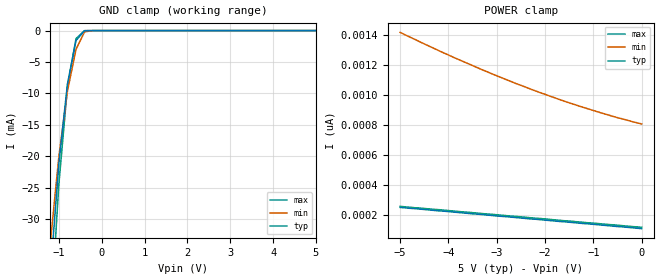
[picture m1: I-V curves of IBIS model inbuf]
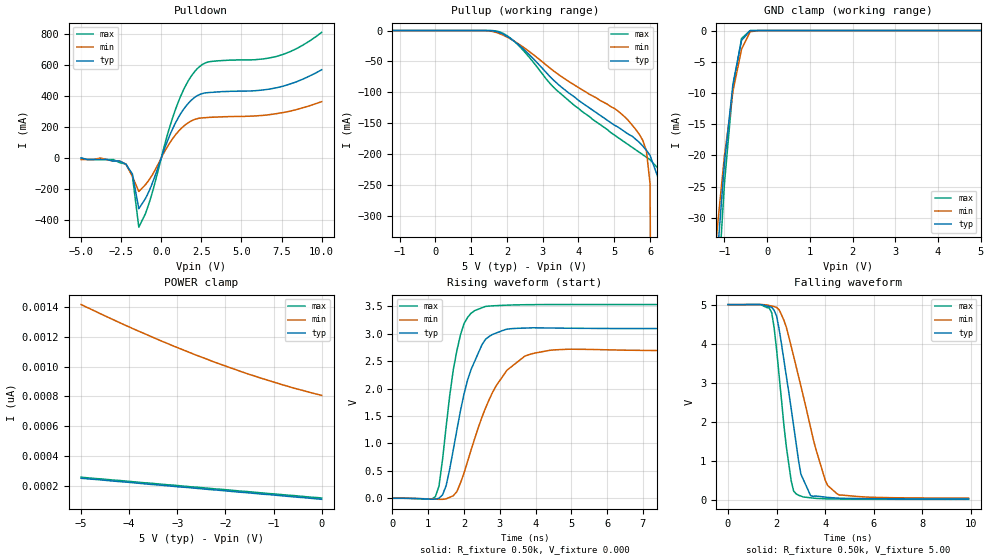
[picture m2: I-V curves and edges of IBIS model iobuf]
| IBIS file 61501n.ibs created by s2ibis2 version 1.0
| North Carolina State University Electronics Research Laboratory  1995
[IBIS ver]   2.1
[File name]   61501n.ibs
[File Rev]   0.1
[Date]   Tuesday, June 10, 1997
[Source]   IDT
[Notes]   1. Temp typ=25C, min=100C, max=0C 2. Ramp rates based on 500
   ohm load
[Copyright]   Copyright 1997, Integrated Device Technology, Inc.
[Disclaimer] Integrated Device Technology, Inc. ("IDT") hereby grants the
   user of this IBIS model a non-exclusive, nontransferable
   license to use this IBIS model under the following terms.
   The user is granted this license only to use the IBIS model
   and is not granted rights to sell, copy (except as needed to
   run the IBIS model), rent, lease or sub-license the IBIS model
   in whole or in part, or in modified form to anyone.
   The User may modify the IBIS model to suit its specific
   applications, but rights to derivative works and such
   modifications shall belong to IDT.
   This IBIS model is provided on an "AS IS" basis and IDT
   makes absolutely no warranty with respect to the information
   contained herein. IDT DISCLAIMS AND CUSTOMER WAIVES ALL
   WARRANTIES, EXPRESS AND IMPLIED, INCLUDING WARRANTIES OF
   MERCHANTABILITY AND FITNESS FOR A PARTICULAR PURPOSE. THE
   ENTIRE RISK AS TO QUALITY AND PERFORMANCE IS WITH THE
   USER ACCORDINGLY, IN NO EVENT SHALL IDT BE LIABLE
   FOR ANY DIRECT OR INDIRECT DAMAGES, WHETHER IN CONTRACT OR
   TORT, INCLUDING ANY LOST PROFITS OR OTHER INCIDENTAL,
   CONSEQUENTIAL, EXEMPLARY, OR PUNITIVE DAMAGES ARISING OUT OF
   THE USE OR APPLICATION OF THE IBIS model.  Further, IDT
   reserves the right to make changes without notice to any
   product herein to improve reliability, function, or design.
   IDT does not convey any license under patent rights or
   any other intellectual property rights, including those of
   third parties. IDT is not obligated to provide maintenance
   or support for the licensed IBIS model.
|   Component IDT54/74FCT16501AT/CT/ET
[Component]   IDT54/74FCT16501AT/CT/ET
[Manufacturer]   Integrated Device Technology Inc.
[Package]
| Following package parameters are for SO56-2(TSSOP) package
|[Package]
|| variable   typ   min   max
|R_pkg   10.00m   9.00m   12.00m
|L_pkg   2.50nH   1.40nH   5.00nH
|C_pkg   0.30pF   0.25pF   0.35pF
| Following package parameters are for SO56-1(SSOP), E56-1(CERPAK) packages
| variable   typ   min   max
R_pkg   15.00m   10.00m   20.00m
L_pkg   3.10nH   1.80nH   6.20nH
C_pkg   0.40pF   0.30pF   0.53pF
[Pin]  signal_name   model_name   R_pin   L_pin   C_pin
1   OEAB   inbuf
2   LEAB   inbuf
3   A1   iobuf
4   GND   GND
5   A2   iobuf
6   A3   iobuf
7   VCC   POWER
8   A4   iobuf
9   A5   iobuf
10   A6   iobuf
11   GND   GND
12   A7   iobuf
13   A8   iobuf
14   A9   iobuf
15   A10   iobuf
16   A11   iobuf
17   A12   iobuf
18   GND   GND
19   A13   iobuf
20   A14   iobuf
21   A15   iobuf
22   VCC   POWER
23   A16   iobuf
24   A17   iobuf
25   GND   GND
26   A18   iobuf
27   OEBAB   inbuf
28   LEBA   inbuf
29   GND   GND
30   CLKBA   inbuf
31   B18   iobuf
32   GND   GND
33   B17   iobuf
34   B16   iobuf
35   VCC   POWER
36   B15   iobuf
37   B14   iobuf
38   B13   iobuf
39   GND   GND
40   B12   iobuf
41   B11   iobuf
42   B10   iobuf
43   B9   iobuf
44   B8   iobuf
45   B7   iobuf
46   GND   GND
47   B6   iobuf
48   B5   iobuf
49   B4   iobuf
50   VCC   POWER
51   B3   iobuf
52   B2   iobuf
53   GND   GND
54   B1   iobuf
55   CLKAB   inbuf
56   GND   GND
| Models and submodels in the file (2): inbuf (Input), iobuf (I/O)
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| in   IN1   dummy_model
| oe   OE1   dummy_model
|   Model inbuf
[Model]   inbuf
Model_type   Input
Vinl =  0.800V
Vinh =  2.000V
C_comp   3.00pF   NA   NA
[Temperature Range]   25.00   100.00   0.000
[Voltage Range]   5.00V   4.50V   5.50V
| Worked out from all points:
|   GND clamp passes 1 mA (typ) near -0.52 V on its own axis
[GND_clamp]
| voltage   I(typ)   I(min)   I(max)
-5V       -94.19A    -89.63A    -95.79A
-1.2V     -38.98mA   -33.85mA   -46.68mA
-1V       -21.15mA   -20.02mA   -24.44mA
-800mV    -8.501mA   -9.67mA    -9.006mA
-600mV    -1.59mA    -2.992mA   -1.281mA
-400mV    -20.6uA    -203uA     -9.215uA
-200mV    -4.67nA    -338nA     -858pA
5V        107pA      849pA      102pA
[POWER_clamp]
| voltage   I(typ)   I(min)   I(max)
-5V       249pA      1.419nA    256pA
-3.9V     218pA      1.253nA    225pA
-3.1V     195pA      1.142nA    203pA
-2.3V     172pA      1.04nA     180pA
-1.7V     155pA      970pA      163pA
-1.3V     144pA      927pA      152pA
-600mV    124pA      858pA      133pA
0V        107pA      807pA      116pA
|   Model iobuf
[Model]   iobuf
Model_type   I/O
Polarity   Non-Inverting
Enable   Active-High
Vinl =  0.800V
Vinh =  2.000V
C_comp   3.00pF   NA   NA
[Temperature Range]   25.00   100.00   0.000
[Voltage Range]   5.00V   4.50V   5.50V
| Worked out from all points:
|   slope of the pulldown table from 0 to 0.75 V, typ, clamps not added: 3.81 ohm
|   GND clamp passes 1 mA (typ) near -0.52 V on its own axis
|   rising waveform, R_fixture 0.50k, V_fixture 0.000: 20-80 % time 658ps typ, 971ps min, 448ps max; typ from 0 V to 3.09 V
|   falling waveform, R_fixture 0.50k, V_fixture 5.00: 20-80 % time 701ps typ, 1.18ns min, 509ps max; typ from 5 V to 0.033 V
[Pulldown]
| voltage   I(typ)   I(min)   I(max)
-5V       0A         -10mA      0A
-2.2V     -40mA      -40mA      -40mA
-1.8V     -103mA     -119mA     -115mA
-1.4V     -327mA     -216mA     -446mA
-700mV    -199mA     -132mA     -272mA
400mV     113mA      75.6mA     156mA
900mV     229mA      151mA      317mA
1.6V      342mA      221mA      482mA
2.2V      399mA      252mA      571mA
3.1V      423mA      262mA      622mA
7.2V      453mA      286mA      655mA
10V       569mA      363mA      810mA
[Pullup]
| voltage   I(typ)   I(min)   I(max)
-5V       0A         0A         0A
1.8V      -3.431mA   -5.195mA   -2.259mA
2.4V      -26.84mA   -24.64mA   -28.63mA
3.4V      -85.43mA   -69.47mA   -97.13mA
5.4V      -168mA     -146mA     -185mA
5.7V      -181mA     -168mA     -197mA
5.9V      -194mA     -195mA     -205mA
6V        -202mA     -247mA     -209mA
6.4V      -266mA     -4.007A    -234mA
6.8V      -4.306A    -13.45A    -282mA
7.2V      -14.25A    -24.15A    -3.045A
10V       -94.19A    -104A      -81.22A
[GND_clamp]
| voltage   I(typ)   I(min)   I(max)
-5V       -94.19A    -89.63A    -95.79A
-1.2V     -38.98mA   -33.85mA   -46.68mA
-1V       -21.15mA   -20.02mA   -24.44mA
-800mV    -8.501mA   -9.67mA    -9.006mA
-600mV    -1.59mA    -2.992mA   -1.281mA
-400mV    -20.6uA    -203uA     -9.215uA
-200mV    -4.67nA    -338nA     -858pA
5V        107pA      849pA      102pA
[POWER_clamp]
| voltage   I(typ)   I(min)   I(max)
-5V       249pA      1.419nA    256pA
-3.9V     218pA      1.253nA    225pA
-3.1V     195pA      1.142nA    203pA
-2.3V     172pA      1.04nA     180pA
-1.7V     155pA      970pA      163pA
-1.3V     144pA      927pA      152pA
-600mV    124pA      858pA      133pA
0V        107pA      807pA      116pA
[Ramp]
| variable   typ   min   max
dV/dt_r   1.86/0.66n   1.61/0.97n   2.12/0.45n
dV/dt_f   2.98/0.70n   2.67/1.07n   3.28/0.53n
R_load = 0.50k
[Rising Waveform]
R_fixture = 0.50k
V_fixture = 0.000
| time   V(typ)   V(min)   V(max)
0s        0V         0V         0V
1.2ns     -15.76mV   -16.29mV   30.79mV
1.3ns     326uV      -19.07mV   222mV
1.5ns     231mV      -10.67mV   1.306V
1.8ns     1.244V     121mV      2.69V
2ns       1.902V     461mV      3.184V
2.3ns     2.501V     1.092V     3.422V
2.9ns     3.013V     2.052V     3.512V
3.8ns     3.105V     2.615V     3.53V
9.9ns     3.094V     2.691V     3.532V
[Falling Waveform]
R_fixture = 0.50k
V_fixture = 5.00
| time   V(typ)   V(min)   V(max)
0s        5V         5V         5V
1.8ns     4.93V      4.962V     4.791V
2ns       4.706V     4.927V     3.853V
2.4ns     3.177V     4.424V     1.374V
2.8ns     1.471V     3.429V     165mV
3ns       667mV      2.918V     106mV
3.4ns     117mV      1.856V     62.57mV
4ns       79.7mV     515mV      36.73mV
4.5ns     54.7mV     158mV      31.45mV
9.9ns     32.64mV    52.28mV    23.2mV
